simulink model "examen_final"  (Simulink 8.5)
settings: Solver=ode45  StartTime=0.0  StopTime=10.0  RelTol=1e-3

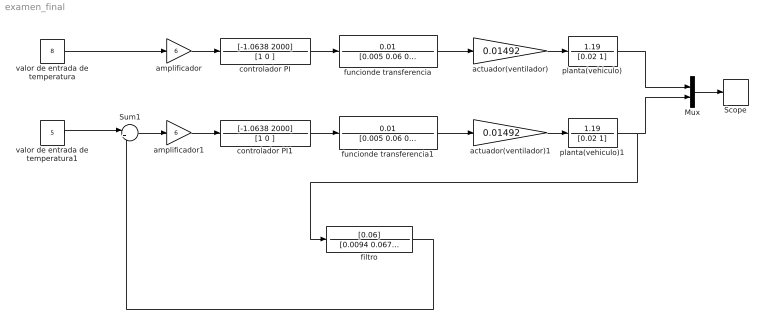
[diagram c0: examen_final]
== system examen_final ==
  Mux : Mux  Inputs=2
  Scope : TimeScope
  Sum1 : Sum  Inputs=|+-
  actuador(ventilador) : Gain  Gain=0.01492
  actuador(ventilador)1 : Gain  Gain=0.01492
  amplificador : Gain  Gain=6
  amplificador1 : Gain  Gain=6
  controlador PI : TransferFcn  Numerator=[-1.0638 2000]  Denominator=[1 0 ]
  controlador PI1 : TransferFcn  Numerator=[-1.0638 2000]  Denominator=[1 0 ]
  filtro : TransferFcn  Numerator=[0.06]  Denominator=[0.0094 0.067 1]
  funcionde transferencia : TransferFcn  Numerator=0.01  Denominator=[0.005 0.06 0.1001]
  funcionde transferencia1 : TransferFcn  Numerator=0.01  Denominator=[0.005 0.06 0.1001]
  planta(vehiculo) : TransferFcn  Numerator=1.19  Denominator=[0.02 1]
  planta(vehiculo)1 : TransferFcn  Numerator=1.19  Denominator=[0.02 1]
  valor de entrada de temperatura : Constant  Value=8
  valor de entrada de temperatura1 : Constant  Value=5
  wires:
  funcionde transferencia/1 -> actuador(ventilador)/1
  actuador(ventilador)/1 -> planta(vehiculo)/1
  valor de entrada de temperatura/1 -> amplificador/1
  controlador PI/1 -> funcionde transferencia/1
  amplificador/1 -> controlador PI/1
  Mux/1 -> Scope/1
  Sum1/1 -> amplificador1/1
  funcionde transferencia1/1 -> actuador(ventilador)1/1
  actuador(ventilador)1/1 -> planta(vehiculo)1/1
  planta(vehiculo)1/1 -> filtro/1, Mux/2
  valor de entrada de temperatura1/1 -> Sum1/1
  controlador PI1/1 -> funcionde transferencia1/1
  amplificador1/1 -> controlador PI1/1
  filtro/1 -> Sum1/2
  planta(vehiculo)/1 -> Mux/1
